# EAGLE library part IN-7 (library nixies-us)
IN-7: large symbol topview nixie tube
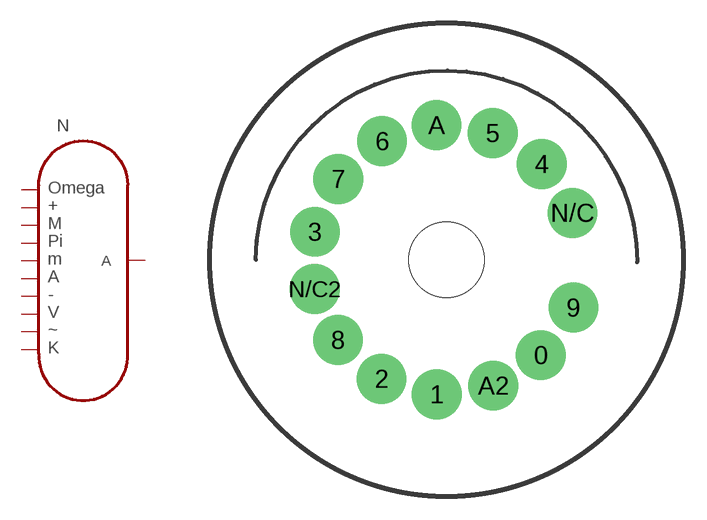
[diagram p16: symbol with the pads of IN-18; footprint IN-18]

Designator prefix N

## IN-7  [IN-18]
0  P$10
1  P$1
3  P$8
4  A
6  P$5
7  P$6
8  P$3
9  P$7
A  P$2
A2  P$9
N/C  P$4

## Footprint IN-18 (pad centres in mm)
May be used with socket: PL31-P
drill 2.3 pad 3.2: 0 6.282,-6.357; 1 -0.645,-8.971; 2 -4.33,-7.938; 3 -8.76,1.863; 4 6.35,6.382; 5 3.09,8.449; 6 -4.291,7.907; 7 -7.214,5.386; 8 -7.228,-5.344; 9 8.456,-3.189; A -0.659,8.976; A2 3.123,-8.394; N/C 8.394,3.123; N/C2 -8.781,-1.948
hole 5 at 0,0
